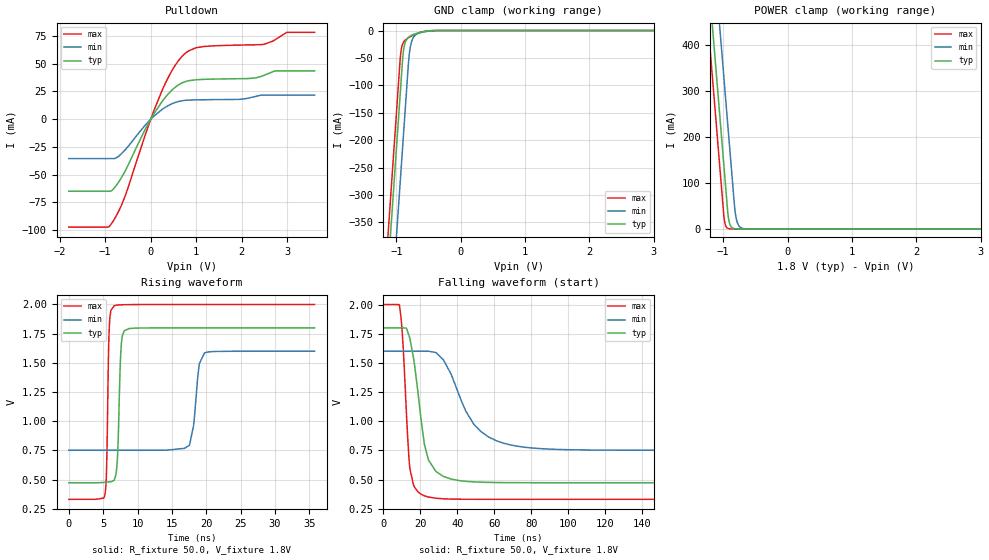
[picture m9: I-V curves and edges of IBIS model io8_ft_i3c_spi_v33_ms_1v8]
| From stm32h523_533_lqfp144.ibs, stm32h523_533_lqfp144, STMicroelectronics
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[Model]   io8_ft_i3c_spi_v33_ms_1v8
Model_type I/O_open_drain
Polarity   Non-Inverting
Enable   Active-Low
| CAP_THRESHOLD on pad IOFT is "UDTCAPC" :
| Rising=20.0% of vddiom   Falling=80.0% of vddiom
| C_comp min and max val. don't necessarily correlate with the min and max pvt
| but are the smallest and greatest pad capacitance found.
| var   typ   min   max
C_comp   3.69208pF  3.66965pF  3.86716pF
|C_comp_pulldown   3.69208pF  3.66965pF  3.86716pF
Vinl = 800.0mV
Vinh = 1.0V
Vmeas = 900.0mV   | Reference voltage for timing measurements
Cref  = 50.0pF   | Timing specification test load capacitance value
Rref  = 1.0MOhm   | Timing specification test load resistance value
Vref  = 990.0mV   | Timing specification test load voltage
[Model Spec]
| TIME_THRESHOLD on pin ZII2CV11 is "CMOS" :
| Rising=40.0% of vdd   Falling=60.0% of vdd
Vinl 693.80000mV 621.80000mV 774.80000mV
Vinh 1.05820V 933.20000mV 1.16320V
| variable   typ   min   max
[Temperature Range] 25.0 125.0 -40.0
| variable   typ   min   max
[Voltage Range] 1.8V 1.6V 2.0V
| variable   typ   min   max
[POWER Clamp Reference] 1.8V 1.6V 2.0V
| variable   typ   min   max
[GND Clamp Reference] 0V 0V 0V
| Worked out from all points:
|   slope of the pulldown table from 0 to 0.27 V, typ, clamps not added: 15.8 ohm
|   GND clamp passes 1 mA (typ) near -0.52 V on its own axis
|   POWER clamp passes 1 mA (typ) near -0.84 V on its own axis
|   rising waveform, R_fixture 50.0, V_fixture 1.8V: 20-80 % time 401ps typ, 855ps min, 285ps max; typ from 0.474 V to 1.8 V
|   falling waveform, R_fixture 50.0, V_fixture 1.8V: 20-80 % time 6.85ns typ, 16.5ns min, 3.35ns max; typ from 1.8 V to 0.474 V
[POWER Clamp]
-1.8V     1.518A     1.709A     1.407A
-1.23V    548.8mA    740.2mA    437.5mA
-1.16V    429.8mA    621.2mA    318.5mA
-1.05V    242.8mA    434.2mA    131.5mA
-980mV    123.8mA    315.2mA    17.95mA
-930mV    38.81mA    230.2mA    1.49mA
-910mV    17.82mA    196.2mA    550.8uA
-890mV    8.18mA     162.2mA    203.5uA
-810mV    363.5uA    33.6mA     3.797uA
-770mV    76.62uA    10.47mA    518.8nA
-710mV    7.416uA    1.822mA    26.34nA
3.6V      0A         0A         0A
[GND Clamp]
-1.8V     -1.579A    -1.74A     -1.515A
-1.24V    -627.3mA   -788.3mA   -562.7mA
-1.05V    -304.3mA   -465.3mA   -239.7mA
-940mV    -117.3mA   -278.3mA   -52.69mA
-930mV    -100.3mA   -261.3mA   -40.52mA
-900mV    -50.11mA   -210.3mA   -24.23mA
-880mV    -30.95mA   -176.3mA   -20.02mA
-810mV    -12.18mA   -57.97mA   -13.23mA
-780mV    -9.807mA   -29.1mA    -11.19mA
-690mV    -5.41mA    -7.142mA   -6.184mA
-420mV    -170.4uA   -446.1uA   -81.94uA
3.6V      5.755nA    953.4nA    228.2pA
| variable   typ   min   max
[Pullup Reference] 1.8V 1.6V 2.0V
| variable   typ   min   max
[Pulldown Reference] 0V 0V 0V
[Pulldown]
-1.8V     -65.02mA   -35.56mA   -97.42mA
-940mV    -65.02mA   -35.56mA   -97.42mA
-850mV    -64.17mA   -35.56mA   -93.49mA
-570mV    -47.32mA   -28.01mA   -70.04mA
-120mV    -9.088mA   -5.279mA   -14.07mA
250mV     16.04mA    8.832mA    26.05mA
520mV     28.19mA    14.82mA    47.53mA
780mV     34.17mA    17.07mA    60.14mA
1.18V     35.97mA    17.56mA    65.65mA
2.49V     39.57mA    21.77mA    67.55mA
2.99V     43.62mA    21.77mA    78.38mA
3.6V      43.62mA    21.77mA    78.38mA
[Ramp]
dV/dt_r 795.76091mV/398.58748ps 508.88166mV/785.35557ps 1.00097V/282.40767ps
dV/dt_f 795.78721mV/6.62413ns 508.97234mV/16.22813ns 1.00099V/3.34704ns
R_load = 50.0
| Removed startup time: 0s 0s 0s  .
| Removed end time: 35.75ns.
[Rising Waveform]
R_fixture   = 50.0
V_fixture   = 1.8V
V_fixture_min = 1.6V
V_fixture_max = 2.0V
0s        473.7mV    751.7mV    331.7mV
5.25ns    477.4mV    751.7mV    371mV
5.5ns     479.2mV    751.7mV    607mV
5.9ns     481.7mV    751.7mV    1.821V
6.6ns     495.2mV    751.7mV    1.989V
7.6ns     1.628V     751.7mV    1.997V
8.05ns    1.774V     751.7mV    1.998V
17.55ns   1.8V       794.9mV    2V
19.75ns   1.8V       1.587V     2V
35.75ns   1.8V       1.6V       2V
| Removed startup time: 0s 0s 0s  .
| Removed end time: 198.75ns.
[Falling Waveform]
R_fixture   = 50.0
V_fixture   = 1.8V
V_fixture_min = 1.6V
V_fixture_max = 2.0V
0s        1.8V       1.6V       2V
8.65ns    1.8V       1.6V       1.995V
10.45ns   1.8V       1.6V       1.695V
14.3ns    1.709V     1.6V       598.4mV
20.3ns    1.022V     1.6V       376.2mV
24.35ns   668.4mV    1.6V       351.2mV
28.4ns    569.6mV    1.589V     340.9mV
48.7ns    481.4mV    979.2mV    332mV
64.9ns    475mV      812.6mV    331.7mV
198.8ns   473.7mV    751.7mV    331.7mV
